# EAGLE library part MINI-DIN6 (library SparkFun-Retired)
Mini DIN 6 Connector SparkFun used to sell this connector and has used it on a couple designs, however the connector and the designs are now retired. Mini DIN 6 Connector [RETIRED] SparkFun Key Counter - PS2 [RETIRED] Commonly found on the back of a computer for PS2 keyboard and mice. Schematic and footprint are proven.
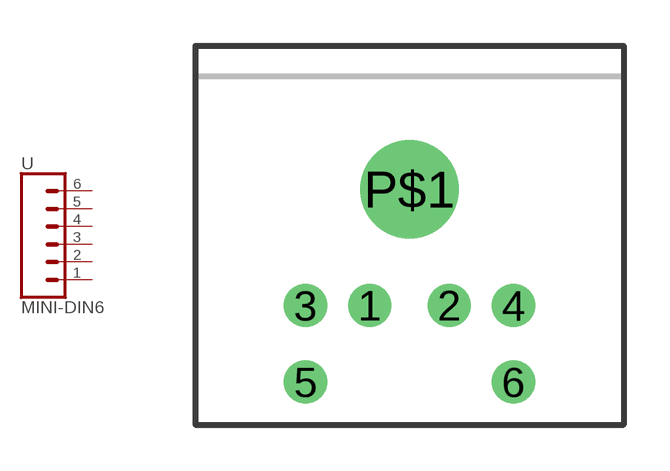
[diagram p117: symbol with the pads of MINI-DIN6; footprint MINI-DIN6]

Designator prefix -

## MINI-DIN6PTH  [MINI-DIN6]
1  1  pas
2  2  pas
3  3  pas
4  4  pas
5  5  pas
6  6  pas

## Footprint MINI-DIN6 (pad centres in mm)
drill 0.9: 1 -1.3,-8.5; 2 1.3,-8.5; 3 -3.4,-8.5; 4 3.4,-8.5; 5 -3.4,-11; 6 3.4,-11
drill 2.2: P$1 0,-4.7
